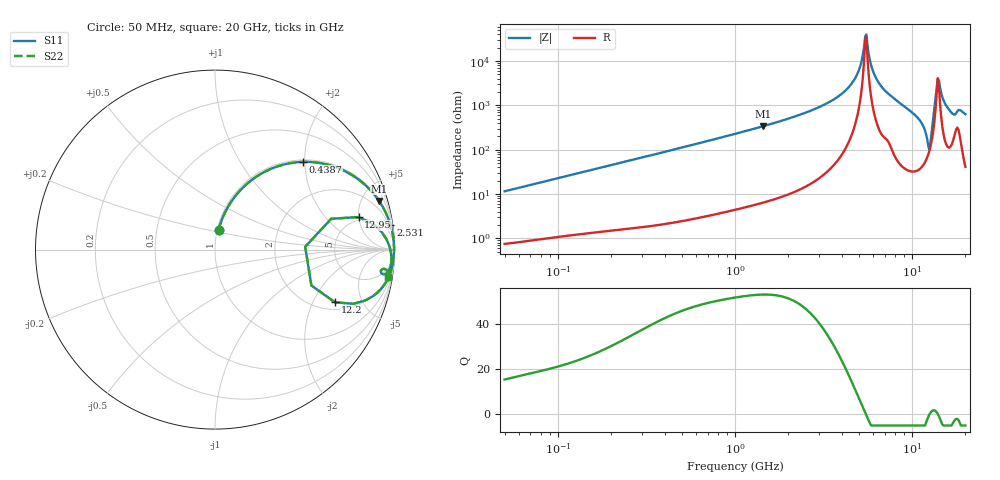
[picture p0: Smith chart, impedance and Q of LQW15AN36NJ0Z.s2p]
!Murata Part Number: LQW15AN36NJ0Z
!These Parameters are Measured in Series Mode Connection
!  o--[Z]--o
!Port1  Port2
!  o-------o
!Freq. Start=50[MHz] Stop=20[GHz], 401[Steps]
# Hz S RI R 50
!Freq.(Hz) S11(Real) S11(Imag) S21(Real) S21(Imag) S12(Real) S12(Imag) S22(Real) S22(Imag)
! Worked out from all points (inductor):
!   401 points, 50 MHz to 20 GHz, reference 50 ohm
!   read as one part in series: L = 36.4 nH near 51.52 MHz
!   highest Q = 53 at 1.433 GHz (marker M1), where L = 37.4 nH
!   self-resonance near 5.434 GHz
!   S11 on the Smith chart (normalised r, x): 50 MHz: 1.01, +0.23; 438.7 MHz: 1.04, +1.96; 2.531 GHz: 1, +14; 12.2 GHz: 2.38, -2.99; 12.95 GHz: 4.49, +4.96; 20 GHz: 2, -13
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5e7  0.0202 0.1118  0.9798 -0.1118  0.9798 -0.1118  0.0202 0.1118
1.364002e8  0.0956 0.2744  0.9044 -0.2744  0.9044 -0.2744  0.0956 0.2744
3.721004e8  0.4102 0.4799  0.5898 -0.4799  0.5898 -0.4799  0.4102 0.4799
4.387496e8  0.4897 0.4887  0.5103 -0.4887  0.5103 -0.4887  0.4897 0.4887
1e9  0.8332 0.3633  0.1668 -0.3633  0.1668 -0.3633  0.8332 0.3633
1.432596e9  0.9145 0.2703  0.0855 -0.2703  0.0855 -0.2703  0.9145 0.2703
2.531158e9  0.9769 0.1398  0.0231 -0.1398  0.0231 -0.1398  0.9769 0.1398
2.728004e9  0.9812 0.1249  0.0188 -0.1249  0.0188 -0.1249  0.9812 0.1249
4.472136e9  0.9965 0.0353  0.00348 -0.0353  0.00348 -0.0353  0.9965 0.0353
4.966507e9  0.9975 0.0172  0.00252 -0.0172  0.00252 -0.0172  0.9975 0.0172
5.352748e9  0.9977 0.00422  0.00227 -0.00422  0.00227 -0.00422  0.9977 0.00422
5.515528e9  0.9977 -0.00103  0.00228 0.00103  0.00228 0.00103  0.9977 -0.00103
6.125241e9  0.9971 -0.0198  0.0029 0.0198  0.0029 0.0198  0.9971 -0.0198
7.442007e9  0.9924 -0.0561  0.00758 0.0561  0.00758 0.0561  0.9924 -0.0561
1.098561e10  0.944 -0.1951  0.056 0.1951  0.056 0.1951  0.944 -0.1951
1.220001e10  0.6681 -0.2937  0.3319 0.2937  0.3319 0.2937  0.6681 -0.2937
1.257102e10  0.5025 0.0157  0.4975 -0.0157  0.4975 -0.0157  0.5025 0.0157
1.295331e10  0.7996 0.1812  0.2004 -0.1812  0.2004 -0.1812  0.7996 0.1812
1.375312e10  0.969 0.0263  0.031 -0.0263  0.031 -0.0263  0.969 0.0263
1.417136e10  0.9801 -0.0177  0.0199 0.0177  0.0199 0.0177  0.9801 -0.0177
1.646126e10  0.962 -0.1269  0.038 0.1269  0.038 0.1269  0.962 -0.1269
2e10  0.9663 -0.1508  0.0337 0.1508  0.0337 0.1508  0.9663 -0.1508
